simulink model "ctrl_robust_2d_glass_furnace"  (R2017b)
settings: Solver=ode45  StartTime=0.0  StopTime=18000  RelTol=1e-3
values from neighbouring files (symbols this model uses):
  w = [196;186;150;145;140;105;85;83;85;80;80]    [readW.m]
undefined symbols (not defined in the file or in its folder): b
libraries: dps x8

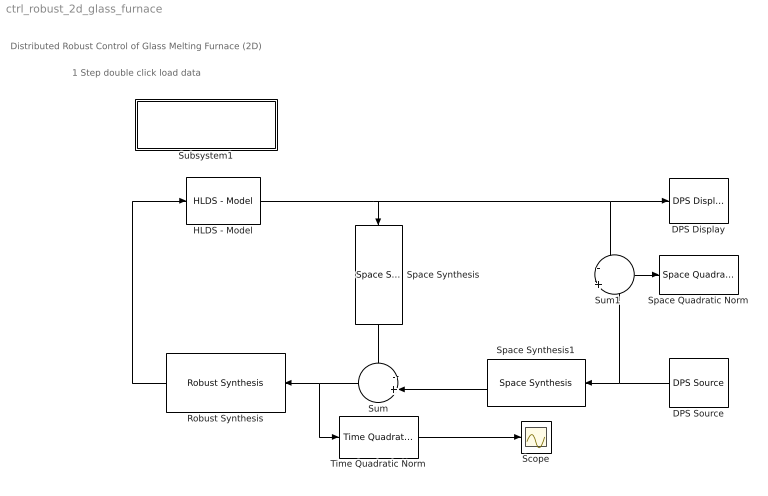
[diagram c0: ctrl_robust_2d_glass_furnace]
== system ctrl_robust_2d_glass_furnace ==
  note: Distributed Robust Control of Glass Melting Furnace (2D)
  note: 1 Step double click load data
  DPS Display : dps/DPS Display  graphType=surf  pointCoord=p'  elementsVar=e  showColor=on  minC=0  maxC=160  showDeform=on  deform=z  deformScale=0.001  showScope=off  responseVar=H  aviparam=0
  DPS Source : dps/DPS Source  equation=0.1*w  responseVar=0  showInput=on  pointsCoord=p'  elementsVar=e  samplePeriod=300
  HLDS - Model : dps/Controlled Systems/HLDS - Model  StepResponse=H  samplePeriod=300  u_step=1
  Robust Synthesis : dps/Temporal Synthesis/Robust Synthesis  b=b  a=a  alfa=[.92;.91;.9;.88]  SamplePeriod=300
  Scope : Scope
  Space Quadratic Norm : dps/Quadratic norms/Space Quadratic Norm  StepResponse=H  showNorm=on
  Space Synthesis : dps/Space Synthesis/Space Synthesis  PCH=H  weights=[]
  Space Synthesis1 : dps/Space Synthesis/Space Synthesis  PCH=H  weights=[]
  Subsystem1 : Subsystem
  Sum : Sum  Inputs=-+|
  Sum1 : Sum  Inputs=-|+
  Time Quadratic Norm : dps/Quadratic norms/Time Quadratic Norm
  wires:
  HLDS - Model/1 -> Space Synthesis/1, Sum1/1, DPS Display/1
  Robust Synthesis/1 -> HLDS - Model/1
  DPS Source/1 -> Sum1/2, Space Synthesis1/1
  Space Synthesis1/1 -> Sum/2
  Space Synthesis/1 -> Sum/1
  Sum/1 -> Time Quadratic Norm/1, Robust Synthesis/1
  Sum1/1 -> Space Quadratic Norm/1
  Time Quadratic Norm/1 -> Scope/1

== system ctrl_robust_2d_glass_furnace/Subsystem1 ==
